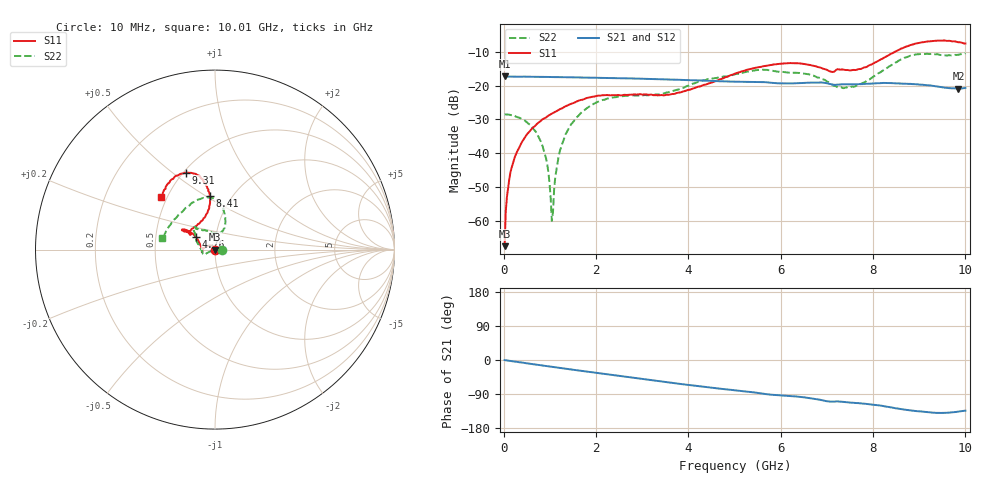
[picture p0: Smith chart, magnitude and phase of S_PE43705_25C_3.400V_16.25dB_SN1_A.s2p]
! Device ID: PE43705
! Serial: 1
! Insertion: A
! Impedance: 50 ohm
! Temp: 25C
! VDD: 3.400V
! Attenuation Step: 16.25dB
#  Hz  S  RI  R  50
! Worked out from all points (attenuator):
!   401 points, 10 MHz to 10.01 GHz, reference 50 ohm
!   highest |S21| = -17.30 dB at 10 MHz (marker M1); lowest = -20.9 dB at 9.86 GHz (marker M2)
!   lowest |S11| = -67.5 dB at 10 MHz (marker M3), VSWR 1.00, Z = 50 + j0.0403 ohm
!   |S11| at or under -10 dB: start of sweep to 8.48 GHz
!   |S22| runs from -60.0 to -10.4 dB; largest |S21 - S12| = 0.0015
!   S11 on the Smith chart (normalised r, x): 10 MHz: 1.00, +0.00; 4.76 GHz: 0.80, +0.12; 8.41 GHz: 0.79, +0.52; 9.31 GHz: 0.51, +0.56; 10.01 GHz: 0.47, +0.33
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1e7  -0.000129 0.000403  0.1364 -0.000553  0.1365 -0.000509  0.0376 2.39e-05
1.1e8  0.000148 0.00407  0.1358 -0.00484  0.1358 -0.00475  0.0372 0.000958
2.6e8  -0.00162 0.00969  0.1351 -0.011  0.1351 -0.011  0.0347 0.00337
5.6e8  -0.00965 0.0191  0.133 -0.0231  0.1331 -0.023  0.0256 0.00611
7.85e8  -0.0194 0.0225  0.1309 -0.0318  0.1309 -0.0316  0.0146 0.00498
9.1e8  -0.0252 0.0225  0.1293 -0.0367  0.1293 -0.0365  0.00776 0.00324
1.035e9  -0.0315 0.0222  0.1273 -0.0413  0.1274 -0.0412  0.000318 0.000948
1.085e9  -0.034 0.0216  0.1266 -0.0429  0.1266 -0.0429  -0.00294 -0.000312
1.16e9  -0.0375 0.0208  0.1257 -0.0456  0.1255 -0.0455  -0.00711 -0.0018
1.26e9  -0.0421 0.0193  0.1238 -0.0493  0.1239 -0.0492  -0.0131 -0.00417
1.685e9  -0.0609 0.00904  0.1156 -0.0635  0.1157 -0.0635  -0.0374 -0.0156
2.285e9  -0.0714 -0.00909  0.1011 -0.081  0.1013 -0.081  -0.0585 -0.0279
3.36e9  -0.0717 -0.00504  0.0695 -0.1032  0.0696 -0.103  -0.0741 -0.00411
4.76e9  -0.1068 0.0725  0.0265 -0.1125  0.0268 -0.1126  -0.1095 0.0812
5.01e9  -0.1225 0.0876  0.0198 -0.1127  0.0199 -0.1127  -0.1137 0.0937
6.685e9  -0.1702 0.1008  -0.0225 -0.1084  -0.0225 -0.1084  -0.0856 0.1123
7.435e9  -0.1148 0.1256  -0.0384 -0.0974  -0.0381 -0.0976  0.00885 0.0938
8.36e9  -0.0266 0.285  -0.0614 -0.0901  -0.0614 -0.0902  0.0557 0.185
8.41e9  -0.0296 0.2969  -0.0628 -0.089  -0.063 -0.0889  0.0534 0.1942
9.31e9  -0.1631 0.4285  -0.0747 -0.0649  -0.0745 -0.0649  -0.1015 0.2749
9.86e9  -0.2755 0.3387  -0.0651 -0.0626  -0.0653 -0.062  -0.2559 0.1287
1.001e10  -0.2982 0.2937  -0.0642 -0.067  -0.0646 -0.067  -0.2947 0.0622
